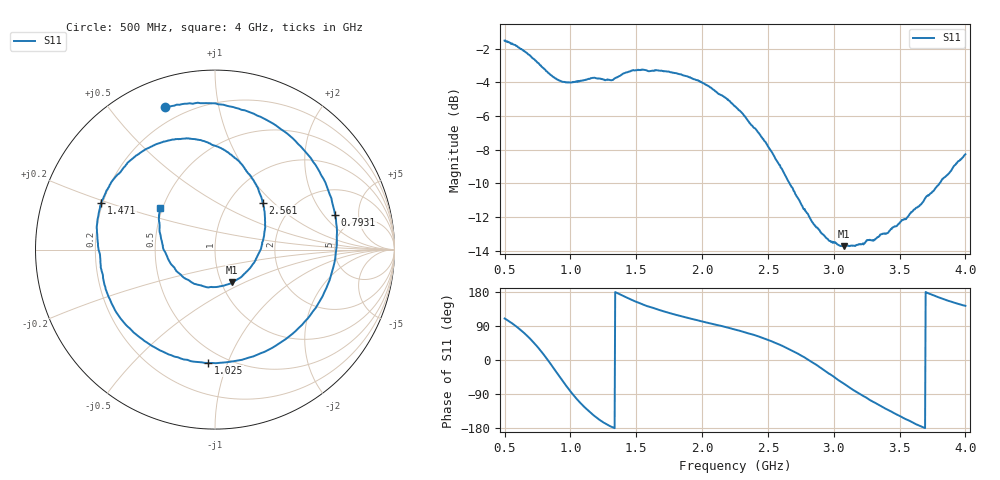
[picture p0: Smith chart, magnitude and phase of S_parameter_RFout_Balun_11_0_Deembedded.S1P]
!Agilent Technologies,E5071B,MY42403504,A.06.51
!Date: Wed Feb 26 14:57:28 2014
!Data & Calibration Information:
!Freq	S11:SOLT1(ON)
# Hz S dB R 50
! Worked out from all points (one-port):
!   801 points, 500 MHz to 4 GHz, reference 50 ohm
!   lowest |S11| = -13.7 dB at 3.077 GHz (marker M1), VSWR 1.52, Z = 56.3 - j21.4 ohm
!   |S11| at or under -10 dB: 2.665 GHz to 3.803 GHz (1.139 GHz wide, 35.2 % of centre)
!   S11 on the Smith chart (normalised r, x): 500 MHz: 0.13, +0.70; 793.1 MHz: 3.51, +2.63; 1.025 GHz: 0.41, -0.86; 1.471 GHz: 0.19, +0.19; 2.561 GHz: 1.42, +0.86; 4 GHz: 0.48, +0.26
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5e8  -1.51 109.5
5.83125e8  -1.78 89.8
6.53125e8  -2.16 69.7
7.23125e8  -2.62 45.3
7.93125e8  -3.14 16.1
8.28125e8  -3.41 -0.1
8.63125e8  -3.64 -17.1
9.375e8  -3.95 -53.7
9.8125e8  -4.00 -74.3
1.025e9  -3.97 -93.4
1.099375e9  -3.88 -121.8
1.178125e9  -3.72 -146.5
1.24375e9  -3.81 -163.3
1.375e9  -3.62 173.5
1.47125e9  -3.29 157.9
1.655e9  -3.27 134.3
1.8125e9  -3.47 118.3
2.03125e9  -4.15 99.1
2.25e9  -5.41 80.2
2.560625e9  -8.57 44.5
2.6875e9  -10.28 23.9
2.915e9  -13.01 -24.1
3.076875e9  -13.73 -62.2
3.125e9  -13.72 -73.7
3.34375e9  -13.14 -118.7
3.5625e9  -11.99 -158.3
3.72e9  -10.72 175.7
4e9  -8.27 142.9
